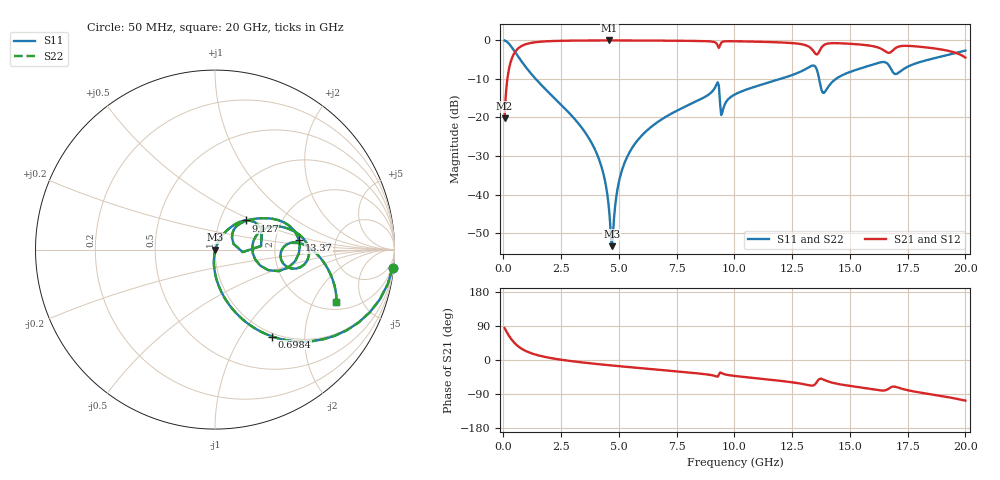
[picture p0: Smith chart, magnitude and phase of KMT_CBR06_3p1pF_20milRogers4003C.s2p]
! Data measured by Modelithics Inc. support@modelithics.com 813-866-6335
! KEMET CBR0603 3.1pF, Pad Width= 0.851mm, Pad Length= 0.64mm, Pad Gap= 0.62mm, 20mil Rogers 4003C substrate Data, January 2022
# hz S ma R 50
! 2 Port Network Data from SP1.SP block
! freq  magS11  angS11  magS21  angS21  magS12  angS12  magS22  angS22
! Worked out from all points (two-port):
!   401 points, 50 MHz to 20 GHz, reference 50 ohm
!   highest |S21| = -0.02 dB at 4.589 GHz (marker M1); lowest = -20.2 dB at 50 MHz (marker M2)
!   |S21| within 3 dB of the highest: 502.9 MHz to 13.45 GHz (12.95 GHz wide, 186 % of centre); 13.66 GHz to 16.59 GHz (2.925 GHz wide, 19.3 % of centre)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
!   lowest |S11| = -53.4 dB at 4.688 GHz (marker M3), VSWR 1.00, Z = 50.2 - j0.0846 ohm
!   |S11| at or under -10 dB: 1.396 GHz to 11.99 GHz (10.6 GHz wide, 158 % of centre); 13.67 GHz to 14.39 GHz (725.6 MHz wide, 5.17 % of centre)
!   |S22| runs from -53.4 to 0.0 dB; largest |S21 - S12| = 0
!   S11 on the Smith chart (normalised r, x): 50 MHz: 1, -20; 698.4 MHz: 0.95, -1.39; 9.127 GHz: 1.32, +0.45; 13.37 GHz: 2.72, +0.37; 20 GHz: 2.38, -3.08
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5e7  0.9952 -5.8  0.09787 84.2  0.09787 84.2  0.9952 -5.8
2.99375e8  0.8605 -31.5  0.5086 58.5  0.5086 58.5  0.8605 -31.5
6.98375e8  0.58 -56.6  0.8136 33.3  0.8136 33.3  0.58 -56.6
1.54625e9  0.2826 -78.1  0.9579 11.6  0.9579 11.6  0.2826 -78.1
3.391625e9  0.07351 -94.9  0.9954 -6.3  0.9954 -6.3  0.07351 -94.9
4.2395e9  0.02322 -96.8  0.9976 -11.8  0.9976 -11.8  0.02322 -96.8
4.588625e9  0.005634 -82.1  0.9977 -13.9  0.9977 -13.9  0.005634 -82.1
4.688375e9  0.002142 -23.2  0.9977 -14.5  0.9977 -14.5  0.002142 -23.2
4.987625e9  0.01411 64.9  0.9975 -16.2  0.9975 -16.2  0.01411 64.9
5.33675e9  0.02996 67.5  0.9971 -18.2  0.9971 -18.2  0.02996 67.5
6.73325e9  0.08961 62.4  0.9931 -25.9  0.9931 -25.9  0.08961 62.4
9.12725e9  0.2353 43.6  0.9519 -41.5  0.9519 -41.5  0.2353 43.6
9.276875e9  0.2856 24.1  0.8566 -43.8  0.8566 -43.8  0.2856 24.1
9.476375e9  0.1169 36.0  0.9563 -35.4  0.9563 -35.4  0.1169 36.0
1.0025e10  0.1995 46.2  0.9739 -42.2  0.9739 -42.2  0.1995 46.2
1.336662e10  0.4704 6.5  0.7624 -67.5  0.7624 -67.5  0.4704 6.5
1.3616e10  0.3729 -18.8  0.6708 -53.7  0.6708 -53.7  0.3729 -18.8
1.386538e10  0.2081 3.1  0.8656 -51.9  0.8656 -51.9  0.2081 3.1
1.531175e10  0.419 16.5  0.89 -71.1  0.89 -71.1  0.419 16.5
1.670825e10  0.4646 -13.2  0.6898 -74.5  0.6898 -74.5  0.4646 -13.2
1.78055e10  0.4974 3.2  0.838 -83.4  0.838 -83.4  0.4974 3.2
2e10  0.7379 -23.5  0.5979 -107.2  0.5979 -107.2  0.7379 -23.5
